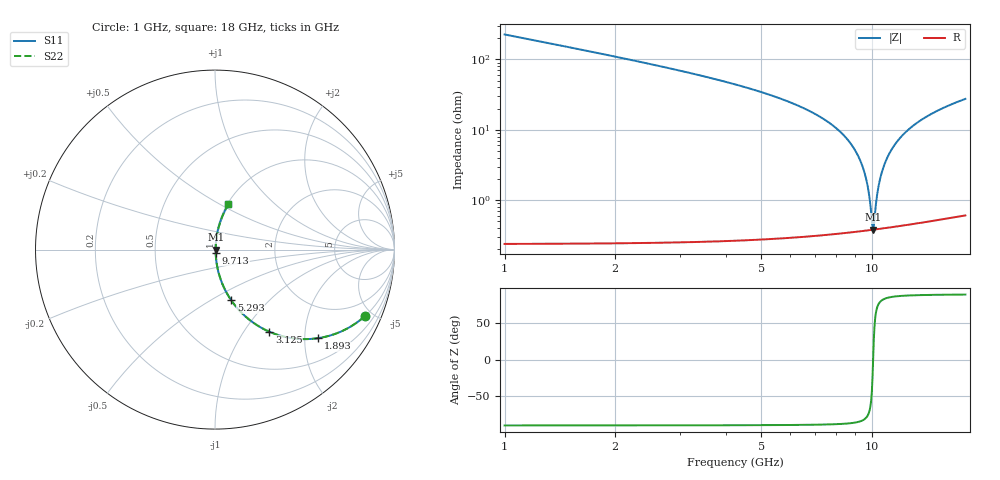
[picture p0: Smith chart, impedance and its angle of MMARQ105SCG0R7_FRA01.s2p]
! MMARQ105SCG0R7_FRA01  S-PARAMETER MODEL  ( General Type )
! Model Generated by TAIYO YUDEN Corporation (http://www.ty-top.com)
! Version 1.0
! TAIYO YUDEN Control No. 200326
! Copyright(c) 2020 TAIYO YUDEN CO.,LTD. All Rights Reserved.
! Product Description (link to TY-COMPAS)
! https://ds.yuden.co.jp/TYCOMPAS/or/detail?pn=MMARQ105SCG0R7BFRA01&u=M
! Products Name : Multilayer Ceramic Capacitors
! Characteristics :
!  Capacitance : 0.7 pF , Rated Voltage : 250V , TCC : CG / C0G
!  Case Size : 1.0 x 0.5 / 0.039 x 0.02 [mm/inch] , Thickness : 0.5 / 0.02 [mm/inch]
!  (Conditions: Temperature = 25 degC , DC Bias Current/Voltage = 0A / 0V)
! External Node Assignments :
!  1  o---| |---o  2
! GND o---------o GND
! Frequency Range : 1GHz  -  18GHz  [ 401 STEP ]
# MHz S RI R 50
! Freq[MHz].  S11 Real  S11 Imag  S21 Real  S21 Imag  S12 Real  S12 Imag  S22 Real  S22 Imag
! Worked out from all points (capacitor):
!   401 points, 1 GHz to 18 GHz, reference 50 ohm
!   read as one part in series: C = 700 fF near 1.085 GHz
!   lowest |Z| = 382 mohm at 10.1 GHz (marker M1)
!   series resonance near 10.09 GHz, so ESL is about 360 pH
!   S11 on the Smith chart (normalised r, x): 1 GHz: 1.00, -4.51; 1.893 GHz: 1.00, -2.32; 3.125 GHz: 1.01, -1.32; 5.293 GHz: 1.01, -0.62; 9.713 GHz: 1.01, -0.03; 18 GHz: 1.01, +0.55
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1000  0.8351 -0.3706  0.1649 0.3706  0.1649 0.3706  0.8351 -0.3706
1892.5  0.5734 -0.4935  0.4266 0.4935  0.4266 0.4935  0.5734 -0.4935
3125  0.3029 -0.4576  0.6971 0.4576  0.6971 0.4576  0.3029 -0.4576
3847.5  0.2045 -0.4008  0.7955 0.4008  0.7955 0.4008  0.2045 -0.4008
5292.5  0.0905 -0.2824  0.9095 0.2824  0.9095 0.2824  0.0905 -0.2824
6695  0.0376 -0.1823  0.9624 0.1823  0.9624 0.1823  0.0376 -0.1823
8480  0.0095 -0.0777  0.9905 0.0777  0.9905 0.0777  0.0095 -0.0777
9075  0.00581 -0.0474  0.9942 0.0474  0.9942 0.0474  0.00581 -0.0474
9500  0.00438 -0.0269  0.9956 0.0269  0.9956 0.0269  0.00438 -0.0269
9712.5  0.00399 -0.0171  0.996 0.0171  0.996 0.0171  0.00399 -0.0171
9840  0.00386 -0.0112  0.9961 0.0112  0.9961 0.0112  0.00386 -0.0112
10010  0.00379 -0.00357  0.9962 0.00357  0.9962 0.00357  0.00379 -0.00357
10095  0.0038 0.000203  0.9962 -0.000203  0.9962 -0.000203  0.0038 0.000203
10180  0.00383 0.00395  0.9962 -0.00395  0.9962 -0.00395  0.00383 0.00395
10307.5  0.00394 0.0095  0.9961 -0.0095  0.9961 -0.0095  0.00394 0.0095
10435  0.00411 0.015  0.9959 -0.015  0.9959 -0.015  0.00411 0.015
10817.5  0.00495 0.031  0.995 -0.031  0.995 -0.031  0.00495 0.031
11455  0.00737 0.0565  0.9926 -0.0565  0.9926 -0.0565  0.00737 0.0565
12347.5  0.0126 0.0898  0.9874 -0.0898  0.9874 -0.0898  0.0126 0.0898
13580  0.0225 0.1318  0.9775 -0.1318  0.9775 -0.1318  0.0225 0.1318
15195  0.0392 0.1807  0.9608 -0.1807  0.9608 -0.1807  0.0392 0.1807
18000  0.0749 0.2523  0.9251 -0.2523  0.9251 -0.2523  0.0749 0.2523
